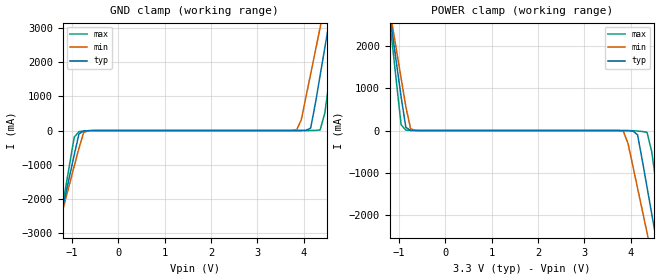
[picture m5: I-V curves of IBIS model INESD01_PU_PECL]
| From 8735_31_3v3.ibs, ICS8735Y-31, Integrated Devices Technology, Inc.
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[Model]   INESD01_PU_PECL
Model_type  Input
Polarity   Non-Inverting
Vinl = 0.8V
Vinh = 2.0V
|   typ   min   max
C_comp   2pF   1.5pF   2.5pF
|   typ   min   max
[Voltage range]  3.3V   3.15V   3.45V
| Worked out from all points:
|   GND clamp passes 1 mA (typ) near -0.55 V on its own axis
|   POWER clamp passes 1 mA (typ) near -0.67 V on its own axis
[GND_clamp]
|Voltage   I(typ)   I(min)   I(max)
-3.3V     -15.3A     -13.19A    -18.82A
-1.361V   -3.24A     -3.145A    -3.432A
-1.259V   -2.606A    -2.617A    -2.622A
-952.6mV  -705.4mA   -1.038A    -192.5mA
-850.5mV  -99.96mA   -513.6mA   -31.29mA
-646.4mV  -3.852mA   -3.611mA   -8.361mA
3.844V    64.83uA    13.07mA    7.183uA
4.151V    73.26mA    1.652A     800.8uA
4.355V    1.607A     3.003A     15.37mA
4.559V    3.233A     4.356A     1.553A
4.763V    4.861A     5.711A     3.635A
6.6V      19.56A     17.94A     22.42A
[POWER_clamp]
|Voltage   I(typ)   I(min)   I(max)
-3.3V     19.56A     16.84A     24.11A
-1.259V   3.233A     3.262A     3.235A
-1.157V   2.419A     2.586A     2.194A
-952.6mV  795.8mA    1.236A     137.7mA
-850.5mV  73.26mA    563.1mA    8.081mA
-646.4mV  471.5uA    1.942mA    367.2uA
3.844V    -890.5uA   -18.21mA   -111uA
4.151V    -99.96mA   -1.362A    -11.88mA
4.355V    -1.338A    -2.415A    -41.77mA
4.559V    -2.606A    -3.47A     -1.313A
4.763V    -3.875A    -4.526A    -2.933A
6.6V      -15.3A     -14.05A    -17.51A
